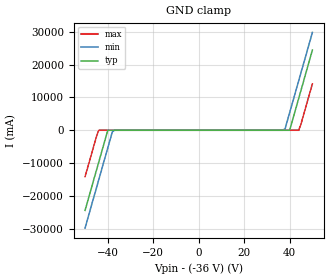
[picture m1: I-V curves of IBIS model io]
| TEXAS INSTRUMENTS INCORPORATED
| 1 Channel Bi-directional ESD-SURGE Protection Device
| Marketing Part #   Voltage Range   Package-type   #pins/pkg drawing
| TSD36C   -36V-36V   SOD-323   2/DYF
[IBIS Ver]   4.1
[Comment char]  |_char
[File Name]   tsd36c.ibs
[File Rev]   1.0
"[Date]   Dec 20, 2023 "
[Source]   Data created from TI-SPICE simulations at TI-SLL/HVL.
   The following is an IBIS list for the ESD851.
   Please contact sllibis@ti.com with questions and
   comments concerning SLL IBIS models.
[Notes]
   - New measurements under nominal conditions only.
[Disclaimer]
"| TI and its licensors and suppliers make no warranties, either expressed"
"| or implied, with respect to this  model, including the warranties of "
"| provided solely on an ""as is"" basis. The entire risk as to its quality "
| and performance is with the customer.
[Copyright]
| (C) Copyright 2023 Texas Instruments Incorporated. All rights reserved.
| Component TSD36C_DYF 2-PIN SOD-323
[Component]   TSD36C_DYF
"[Manufacturer]   Texas Instruments, Inc."
[Package]   |2 SOD-323 - DYF package
   typ   min   max
R_pkg   34.0E-03   27.2E-03   40.8E-03
L_pkg   3.8E-10   3.04E-10   4.56E-10
C_pkg   5.7E-13   4.5E-13   6.8E-13
[Pin]   signal_name   model_name   R_pin   L_pin   C_pin
1   IO   io   2.07E-03   2.09E-10   6.95E-14
2   IO   io   2.07E-03   2.09E-10   6.95E-14
3   GND   gnd   2.07E-03   2.09E-10   6.95E-14
| Models and submodels in the file (1): io (Input)
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|   io Model
[Model]   io
Model_type  Input
| variable   typ   min   max
C_comp   4.3pF   3.5pF   5pF
[Voltage Range]   72   68   76
[Temperature Range]   27   -55   150
[Power Clamp Reference]   0   0   0
[GND Clamp Reference]   -36   -34   -38
[GND Clamp]
|	Voltage  I(typ)   I(min)   I(max)
-50V      -24.4A     -29.8A     -14.1A
-45V      -12.2A     -17.6A     -1.95A
-44V      -9.76A     -15.1A     -5.5nA
-40V      -5nA       -5.37A     -5nA
-38V      -4.75nA    -488mA     -4.75nA
-37V      -4.63nA    -4.63nA    -4.63nA
37V       4.63nA     4.63nA     4.63nA
38V       4.75nA     488mA      4.75nA
40V       5nA        5.37A      5nA
44V       9.76A      15.1A      5.5nA
45V       12.2A      17.6A      1.95A
50V       24.4A      29.8A      14.1A
[Power Clamp]
|   Voltage   I(typ)   I(min)   I(max)
-36V      0A         0A         0A
0V        0A         0A         0A
36V       0A         0A         0A
